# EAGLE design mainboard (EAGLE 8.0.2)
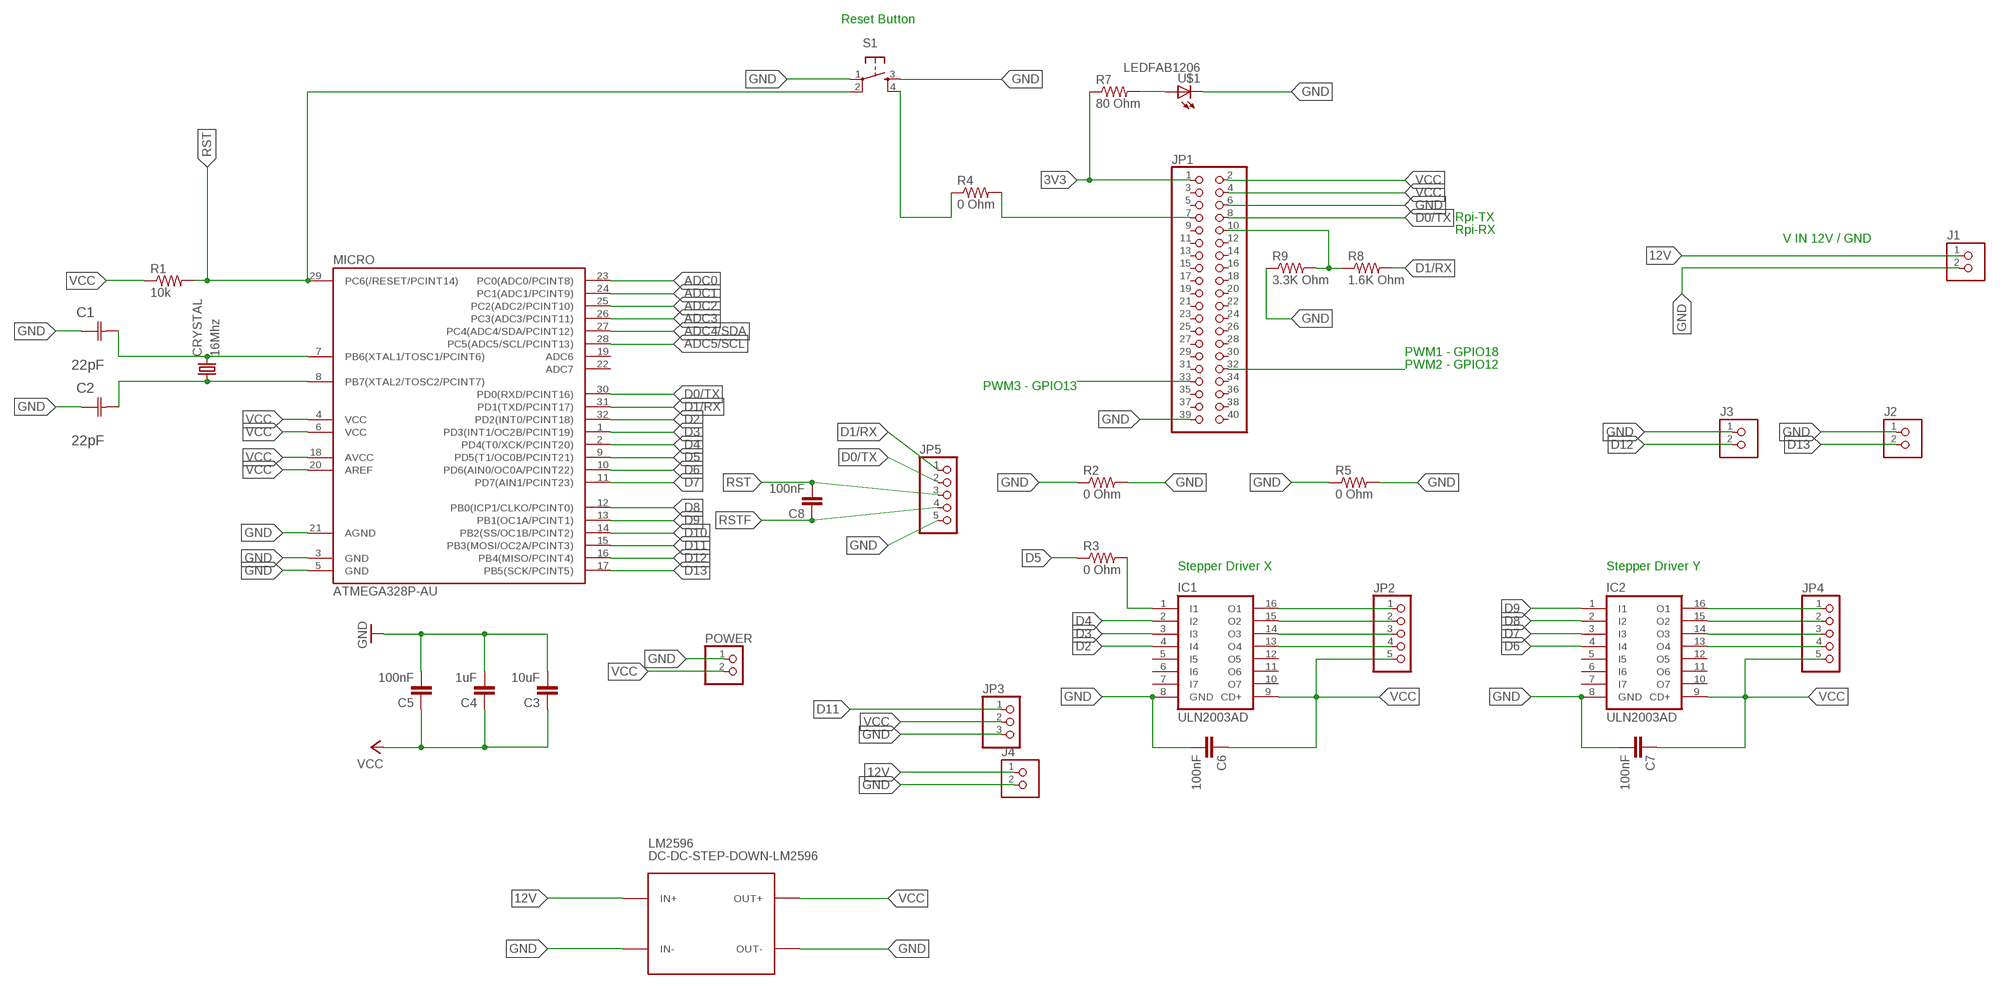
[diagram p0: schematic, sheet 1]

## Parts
C1  22pF  0612ZC225MAT2A  [CAPC3216X178N]
C2  22pF  0612ZC225MAT2A  [CAPC3216X178N]
C3  10uF  CAP1206  [1206]
C4  1uF  CAP1206  [1206]
C5  100nF  CAP1206  [1206]
C6  100nF  CAP1206  [1206]
C7  100nF  CAP1206  [1206]
C8  100nF  CAP1206  [1206]
CRYSTAL  16Mhz  CSM-7X-DU  [CSM-7X-DU]
IC1  ULN2003AD  [SO16]
IC2  ULN2003AD  [SO16]
J1  TERM-1X02-FABLAB  [ED555DS-2DS]
J2  TERM-1X02-FABLAB  [ED555DS-2DS]
J3  TERM-1X02-FABLAB  [ED555DS-2DS]
J4  TERM-1X02-FABLAB  [ED555DS-2DS]
JP1  PINHD-2X20  [2X20]
JP2  PINHD-1X5  [1X05]
JP3  PINHD-1X3  [1X03]
JP4  PINHD-1X5  [1X05]
JP5  PINHD-1X5  [1X05]
LM2596  DC-DC-STEP-DOWN-LM2596  [DC-DC-STEP-DOWN-LM2596]
MICRO  ATMEGA328P-AU  ATMEGA48/88/168-AU  [TQFP32-08]
POWER  PINHD-1X2  [1X02]
R1  10k  RESISTOR1206  [1206]
R2  0 Ohm  RES-US1206FAB  [R1206FAB]
R3  0 Ohm  RES-US1206FAB  [R1206FAB]
R4  0 Ohm  RES-US1206FAB  [R1206FAB]
R5  0 Ohm  RES-US1206FAB  [R1206FAB]
R7  80 Ohm  RES-US1206FAB  [R1206FAB]
R8  1.6K Ohm  RES-US1206FAB  [R1206FAB]
R9  3.3K Ohm  RES-US1206FAB  [R1206FAB]
S1  6MM_SWITCH6MM_SWITCH  [6MM_SWITCH]
U$1  LEDFAB1206  [LED1206FAB]

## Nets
3V3: JP1.1 R7.1
12V: J1.1 J4.1 LM2596.IN+
ADC0: MICRO.23(PC0(ADC0/PCINT8))
ADC1: MICRO.24(PC1(ADC1/PCINT9))
ADC2: MICRO.25(PC2(ADC2/PCINT10))
ADC3: MICRO.26(PC3(ADC3/PCINT11))
ADC4/SDA: MICRO.27(PC4(ADC4/SDA/PCINT12))
ADC5/SCL: MICRO.28(PC5(ADC5/SCL/PCINT13))
D0/TX: JP1.8 JP5.2 MICRO.30(PD0(RXD/PCINT16))
D1/RX: JP5.1 MICRO.31(PD1(TXD/PCINT17)) R8.2
D2: IC1.4(I4) MICRO.32(PD2(INT0/PCINT18))
D3: IC1.3(I3) MICRO.1(PD3(INT1/OC2B/PCINT19))
D4: IC1.2(I2) MICRO.2(PD4(T0/XCK/PCINT20))
D5: IC1.1(I1) MICRO.9(PD5(T1/OC0B/PCINT21)) R3.1 R3.2
D6: IC2.4(I4) MICRO.10(PD6(AIN0/OC0A/PCINT22))
D7: IC2.3(I3) MICRO.11(PD7(AIN1/PCINT23))
D8: IC2.2(I2) MICRO.12(PB0(ICP1/CLKO/PCINT0))
D9: IC2.1(I1) MICRO.13(PB1(OC1A/PCINT1))
D10: MICRO.14(PB2(SS/OC1B/PCINT2))
D11: JP3.1 MICRO.15(PB3(MOSI/OC2A/PCINT3))
D12: J3.2 MICRO.16(PB4(MISO/PCINT4))
D13: J2.2 MICRO.17(PB5(SCK/PCINT5))
GND: C1.1(C1) C2.1(C1) C3.2 C4.2 C5.2 C6.2 C7.2 IC1.8(GND) IC2.8(GND) J1.2 J2.1 J3.1 J4.2 JP1.6 JP1.39 JP3.3 JP5.5 LM2596.IN- LM2596.OUT- MICRO.3(GND) MICRO.5(GND) MICRO.21(AGND) POWER.1 R2.1 R2.2 R5.1 R5.2 R9.1 S1.1(P) U$1.2(C)
N$1: R7.2 U$1.1(A)
N$2: C1.2(C2) CRYSTAL.2 MICRO.7(PB6(XTAL1/TOSC1/PCINT6))
N$3: R4.1 S1.4(S1)
N$7: JP1.10 R8.1 R9.2
N$9: C2.2(C2) CRYSTAL.1 MICRO.8(PB7(XTAL2/TOSC2/PCINT7))
N$10: JP1.32
N$11: JP1.33
N$12: JP1.7 R4.2
N$13: IC1.16(O1) JP2.1
N$14: IC1.15(O2) JP2.2
N$15: IC1.14(O3) JP2.3
N$16: IC1.13(O4) JP2.4
N$17: S1.3(S)
N$25: IC2.16(O1) JP4.1
N$26: IC2.15(O2) JP4.2
N$27: IC2.14(O3) JP4.3
N$28: IC2.13(O4) JP4.4
RST: C8.2 JP5.3 MICRO.29(PC6(/RESET/PCINT14)) R1.2 S1.2(P1)
RSTF: C8.1 JP5.4
VCC: C3.1 C4.1 C5.1 C6.1 C7.1 IC1.9(CD+) IC2.9(CD+) JP1.2 JP1.4 JP2.5 JP3.2 JP4.5 LM2596.OUT+ MICRO.4(VCC) MICRO.6(VCC) MICRO.18(AVCC) MICRO.20(AREF) POWER.2 R1.1
Unconnected: IC1.5(I5) IC1.6(I6) IC1.7(I7) IC1.10(O7) IC1.11(O6) IC1.12(O5) IC2.5(I5) IC2.6(I6) IC2.7(I7) IC2.10(O7) IC2.11(O6) IC2.12(O5) JP1.3 JP1.5 JP1.9 JP1.11 JP1.12 JP1.13 JP1.14 JP1.15 JP1.16 JP1.17 JP1.18 JP1.19 JP1.20 JP1.21 JP1.22 JP1.23 JP1.24 JP1.25 JP1.26 JP1.27 JP1.28 JP1.29 JP1.30 JP1.31 JP1.34 JP1.35 JP1.36 JP1.37 JP1.38 JP1.40 MICRO.19(ADC6) MICRO.22(ADC7)

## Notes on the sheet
- Reset Button
- Rpi-TX
- Rpi-RX
- V IN 12V / GND
- PWM1 - GPIO18
- PWM2 - GPIO12
- PWM3 - GPIO13
- Stepper Driver X | Stepper Driver Y

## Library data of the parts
C1 C2 = AVX_By_element14_Batch_1:0612ZC225MAT2A: Capacitor 1206; MPN: 0612ZC225MAT2A; OC_FARNELL: -; OC_NEWARK: 12N3209; SUPPLIER: AVX; TOLERANCE: ±20%; VALUE: 2.2µF; VOLTAGERATING: 10V
C3-C8 = 01_SparkFun:CAP: Capacitor
CRYSTAL = 01_FAB_Hello:CSM-7X-DU: SMD CRYSTAL; OC_FARNELL: unknown; OC_NEWARK: unknown
IC1 IC2 = uln-udn:ULN2003A: DRIVER ARRAY
J1-J3 = fab:TERM-1X02: 3.5mm terminal block, 2 positions ED555-2DS as found in the fablab inventory.
J4 = fab-modd:TERM-1X02: 3.5mm terminal block, 2 positions ED555-2DS as found in the fablab inventory.
JP1 = pinhead:PINHD-2X20: PIN HEADER
JP2 JP4 JP5 = pinhead:PINHD-1X5: PIN HEADER
JP3 = pinhead:PINHD-1X3: PIN HEADER
LM2596 = diy-modules:DC-DC-STEP-DOWN-LM2596: DC/DC Step-Down Regulator based on LM2596-ADJ chip LM2596 datasheet available here: http://www.ti.com/lit/ds/symlink/lm2596.pdf Click here to find device on ebay.com
MICRO = atmega8:ATMEGA48/88/168
POWER = pinhead:PINHD-1X2: PIN HEADER
R1 = 01_SparkFun:RESISTOR: Resistor
R2-R5 R7-R9 = fab:RES-US: Resistor (US Symbol)
S1 = fab:6MM_SWITCH: OMRON SWITCH
U$1 = fab:LED: LED

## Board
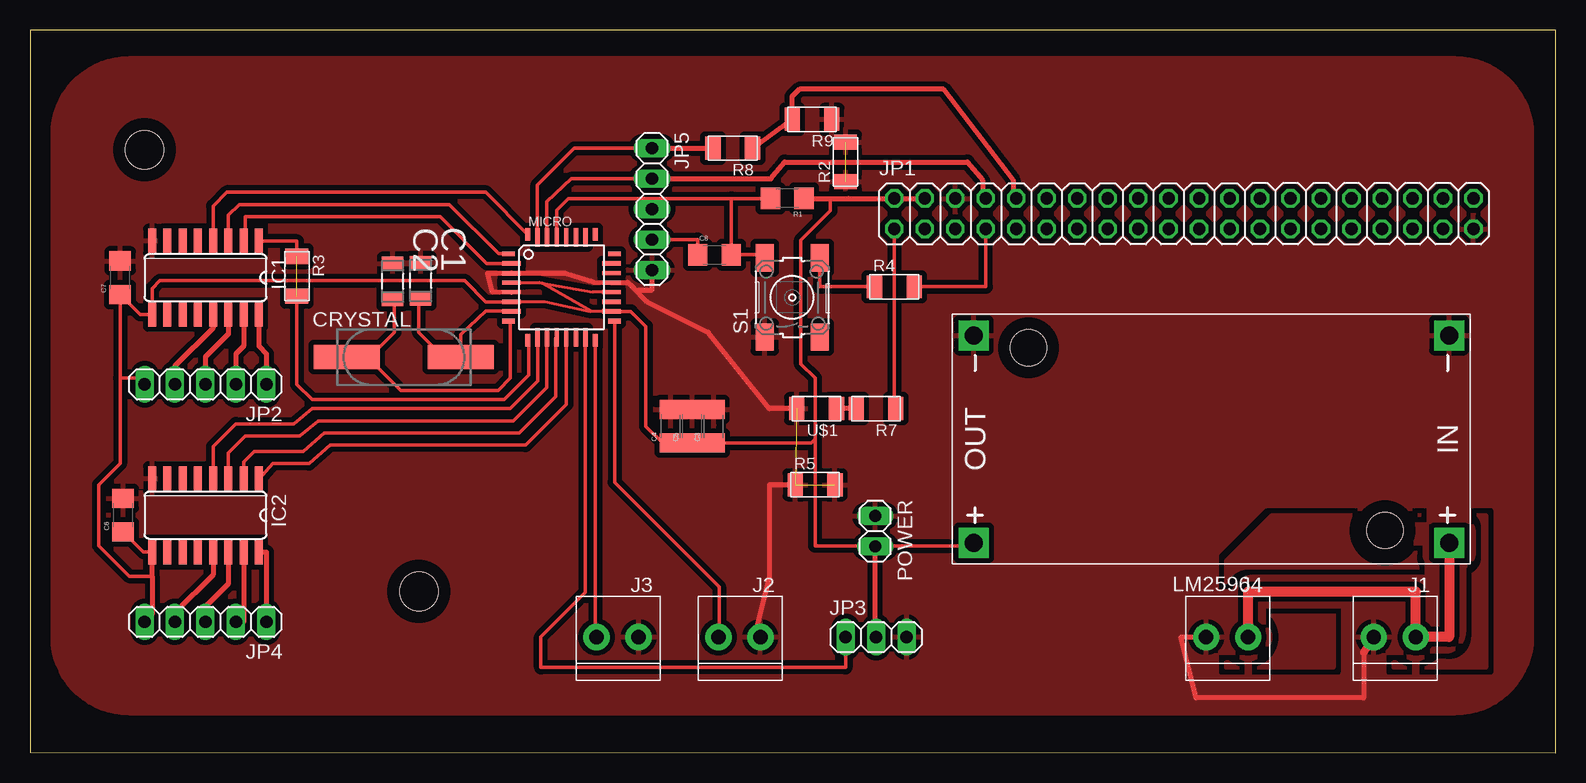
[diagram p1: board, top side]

Size 127.15 x 60.26 mm. Coordinates in mm from the lower left corner, seen from the top.
Outline: 0,0.04 127.15,0 127.15,60.26 0,60.22 0,0.04
Copper layers (1*16): Top 0.035mm / dielectric 1.5mm / Bottom 0.035mm
Design rules "default *": minimum track width 10mil, minimum drill 24mil, track to track 8mil, track to pad 8mil, pad to pad 8mil, via to via 8mil, smd to smd 8mil, copper to edge 40mil, drill to drill 8mil, minimum pad ring 10mil, minimum via ring 8mil, stop-mask expansion 4mil, vias tented up to drill 0mil, thermal gap 16mil
Holes 3.2 mm at 9.54,50.28 32.4,13.45

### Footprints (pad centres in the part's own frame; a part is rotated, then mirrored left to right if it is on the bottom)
CAPC3216X178N = smd 1.118 x 1.803: 1 -1.499,0; 2 1.499,0
1206 = smd 1.6 x 1.8: 1 -1.4,0; 2 1.4,0
CSM-7X-DU = smd 5.5 x 2: 1 -4.75,0; 2 4.75,0
SO16 = smd 0.66 x 2.032: 1 -4.445,-3.073; 2 -3.175,-3.073; 3 -1.905,-3.073; 4 -0.635,-3.073; 5 0.635,-3.073; 6 1.905,-3.073; 7 3.175,-3.073; 8 4.445,-3.073; 9 4.445,3.073; 10 3.175,3.073; 11 1.905,3.073; 12 0.635,3.073; 13 -0.635,3.073; 14 -1.905,3.073; 15 -3.175,3.073; 16 -4.445,3.073
ED555DS-2DS = drill 1.2 pad 2.184: 1 1.8,0; 2 -1.7,0
2X20 = drill 1.016 octagon: 1 -24.13,-1.27; 2 -24.13,1.27; 3 -21.59,-1.27; 4 -21.59,1.27; 5 -19.05,-1.27; 6 -19.05,1.27; 7 -16.51,-1.27; 8 -16.51,1.27; 9 -13.97,-1.27; 10 -13.97,1.27; 11 -11.43,-1.27; 12 -11.43,1.27; 13 -8.89,-1.27; 14 -8.89,1.27; 15 -6.35,-1.27; 16 -6.35,1.27; 17 -3.81,-1.27; 18 -3.81,1.27; 19 -1.27,-1.27; 20 -1.27,1.27; 21 1.27,-1.27; 22 1.27,1.27; 23 3.81,-1.27; 24 3.81,1.27; 25 6.35,-1.27; 26 6.35,1.27; 27 8.89,-1.27; 28 8.89,1.27; 29 11.43,-1.27; 30 11.43,1.27; 31 13.97,-1.27; 32 13.97,1.27; 33 16.51,-1.27; 34 16.51,1.27; 35 19.05,-1.27; 36 19.05,1.27; 37 21.59,-1.27; 38 21.59,1.27; 39 24.13,-1.27; 40 24.13,1.27
1X05 = drill 1.016 long: 1 -5.08,0; 2 -2.54,0; 3 0,0; 4 2.54,0; 5 5.08,0
1X03 = drill 1.016 long: 1 -2.54,0; 2 0,0; 3 2.54,0
DC-DC-STEP-DOWN-LM2596 = drill 1.5 pad 2.5 square: IN+ -19.812,8.636; IN- -19.812,-8.636; OUT+ 19.812,8.636; OUT- 19.812,-8.636 | hole 3: -14.478,7.62; 15.24,-7.62
TQFP32-08 = smd 1.016 x 0.406: 1 -4.42,2.8; 8 -4.42,-2.8; 17 4.42,-2.8; 24 4.42,2.8 | smd 1.524 x 0.356: 2 -4.166,2; 3 -4.166,1.2; 4 -4.166,0.4; 5 -4.166,-0.4; 6 -4.166,-1.2; 7 -4.166,-2; 18 4.166,-2; 19 4.166,-1.2; 20 4.166,-0.4; 21 4.166,0.4; 22 4.166,1.2; 23 4.166,2 | smd 0.406 x 1.016: 9 -2.8,-4.42; 16 2.8,-4.42; 25 2.8,4.42; 32 -2.8,4.42 | smd 0.356 x 1.524: 10 -2,-4.166; 11 -1.2,-4.166; 12 -0.4,-4.166; 13 0.4,-4.166; 14 1.2,-4.166; 15 2,-4.166; 26 2,4.166; 27 1.2,4.166; 28 0.4,4.166; 29 -0.4,4.166; 30 -1.2,4.166; 31 -2,4.166
1X02 = drill 1.016 long: 1 -1.27,0; 2 1.27,0
R1206FAB = smd 1.27 x 1.905: 1 -1.651,0; 2 1.651,0
6MM_SWITCH = smd 2.286 x 1.524: 1 -3.302,2.286; 2 3.302,2.286; 3 -3.302,-2.286; 4 3.302,-2.286
LED1206FAB = smd 1.27 x 1.905: 1 -1.651,0; 2 1.651,0

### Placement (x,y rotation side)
C1  32.55,39.36 270 top
C2  30.22,39.31 270 top
C3  56.99,27.22 90 top
C4  53.38,27.22 90 top
C5  55.19,27.22 90 top
C6  7.76,19.8 90 top
C7  7.51,39.61 90 top
C8  57.04,41.52 0 top
CRYSTAL  31.16,32.98 0 top
IC1  14.62,39.61 180 top
IC2  14.62,19.8 180 top
J1  113.68,9.64 0 top
J2  59.07,9.64 0 top
J3  48.91,9.64 0 top
J4  99.71,9.64 0 top
JP1  96.16,44.95 0 top
JP2  14.62,30.72 180 top
JP3  70.5,9.64 0 top
JP4  14.62,10.91 180 top
JP5  51.83,45.33 270 top
LM2596  98.44,26.15 180 top
MICRO  44.29,38.8 0 top
POWER  70.43,18.47 270 top
R1  63.1,46.22 180 top
R2  67.96,49.26 90 top
R3  22.24,39.74 270 top
R4  72.03,38.85 0 top
R5  65.42,22.34 0 top
R7  70.5,28.69 180 top
R8  58.56,50.41 180 top
R9  65.17,52.82 180 top
S1  63.52,37.96 90 top
U$1  65.55,28.69 180 top

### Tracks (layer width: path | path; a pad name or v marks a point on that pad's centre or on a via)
3V3
  Top 0.305: JP1.1 72.03,28.82 R7.1
12V
  Top 0.813: LM2596.IN+ 118.25,9.64 J1.1 115.48,13.45 101.51,13.45 J4.1
D0/TX
  Top 0.305: JP5.2 45.1,47.87 43.07,45.96 43.07,42.99 MICRO.30 | 51.96,47.87 52.72,48.37 52.21,47.87 51.96,47.87
  Top 0.406: JP5.2 51.96,47.87 61.74,47.87 62.88,49.26 78.12,49.26 79.39,47.74 79.39,46.47 JP1.8
D1/RX
  Top 0.305: MICRO.31 42.29,47.34 45.36,50.41 51.45,50.41 | 51.45,50.41 52.72,50.03 52.34,50.41 JP5.1 51.45,50.41
  Top 0.406: JP5.1 R8.2
D2
  Top 0.305: MICRO.32 37.99,46.72 16.4,46.72 15.26,45.58 IC1.4
D3
  Top 0.305: IC1.3 16.53,44.82 17.42,45.71 34.94,45.71 39.05,41.6 MICRO.1
D4
  Top 0.305: MICRO.2 38.07,40.8 34.18,44.69 17.92,44.69 17.92,42.81 IC1.2
D5  (1 unrouted)
  Top 0.305: R3.1 22.24,42.66 19.09,42.66 IC1.1 | R3.2 22.24,30.72 23.51,29.45 39.51,29.45 41.55,31.48 41.55,34.32 MICRO.9
D6
  Top 0.305: IC2.4 15.26,25.51 17.16,27.42 21.99,27.42 23.51,28.69 40.02,28.69 42.31,30.98 42.31,34.62 MICRO.10
D7
  Top 0.305: IC2.3 16.53,25.01 17.92,26.4 22.5,26.4 24.02,27.67 40.28,27.67 43.07,30.47 43.07,34.62 MICRO.11
D8
  Top 0.305: IC2.2 17.8,24.24 18.69,25.13 22.75,25.13 24.53,26.66 40.78,26.66 43.83,29.71 43.83,34.58 MICRO.12
D9
  Top 0.305: IC2.1 19.09,22.85 20.21,24.12 23.26,24.12 25.04,25.64 41.29,25.64 44.69,29.04 MICRO.13
D11
  Top 0.305: MICRO.15 46.29,13.37 42.56,9.64 42.56,7.1 67.96,7.1 JP3.1
D12
  Top 0.305: MICRO.16 47.09,9.76 J3.2
D13
  Top 0.305: MICRO.17 48.71,22.54 57.42,13.83 57.42,9.69 J2.2
GND  (3 unrouted)
  Top 0.305: MICRO.21 | C4.2 C5.2 C3.2
  Top 0.406: MICRO.5 38.5,38.47 38.12,39.99 MICRO.3 44.59,39.99 47.01,39.23 MICRO.21 | MICRO.21 49.8,39.23 49.87,39.17 | 50.18,38.85 49.87,39.17 | 50.18,38.85 50.44,38.6 51.83,38.6 JP5.5 | 111.14,8.37 111.14,4.56 97.17,4.56 95.9,9.64 J4.2 | MICRO.21 49.87,39.17 | U$1.2 61.61,28.69 56.53,35.04 51.45,37.58 50.18,38.85 | R5.1 61.61,22.34 61.61,14.72 60.34,9.64 61.61,9.64
  Top 0.61: J1.2 111.14,8.37
  pour Top (isolate 0.432, rank 3): 118.76,3.29 8.27,3.29 arc-90 1.92,9.64 1.92,51.55 arc-90 8.27,57.9 118.76,57.9 arc-90 125.11,51.55 125.11,9.64 arc-90
N$1
  Top 0.406: R7.2 U$1.1
N$2
  Top 0.305: C1.2 32.4,37.58 32.4,35.04 34.59,32.85 CRYSTAL.2 35.91,34.87 37.99,36.82 40.11,36.82 MICRO.7
N$3
  Top 0.305: S1.4 65.8,38.85 R4.1
N$7
  Top 0.406: R8.1 R9.2 63.52,54.72 64.15,55.36 76.09,55.36 81.93,47.74 81.93,46.47 JP1.10
N$9
  Top 0.305: C2.2 30.37,37.53 30.37,35.04 28.18,32.85 CRYSTAL.1 28.24,32.85 30.88,30.21 39.01,30.21 40.02,31.23 40.02,35.85 MICRO.8
N$12
  Top 0.305: JP1.7 79.65,38.85 R4.2
N$13
  Top 0.406: IC1.16 19.07,33.9 19.7,33.26 JP2.1
N$14
  Top 0.406: IC1.15 17.8,33.9 17.16,33.26 JP2.2
N$15
  Top 0.406: IC1.14 16.53,34.91 14.62,33.01 JP2.3
N$16
  Top 0.406: IC1.13 15.26,35.42 12.08,32.25 JP2.4
N$18
  pour Top (isolate 1.422, rank 2, no thermals): 99.71,7.1 99.71,15.99 103.52,19.8 121.3,19.8 121.3,7.1 113.68,7.1 113.68,12.18 108.6,12.18 108.6,7.1
N$25
  Top 0.406: IC2.16 19.7,16.73 JP4.1
N$26
  Top 0.406: IC2.15 17.8,10.91 JP4.2
N$27
  Top 0.406: IC2.14 16.53,14.08 14.62,12.18 JP4.3
N$28
  Top 0.406: IC2.13 15.26,14.85 12.08,11.67 JP4.4
RST
  Top 0.305: MICRO.29 43.89,45.26 44.85,46.22 50.94,46.22 | 52.72,46.22 50.94,46.22 | 50.94,46.22 JP5.3 52.72,46.22 | S1.2 60.98,41.52 C8.2 58.44,46.22 | 52.72,46.22 58.44,46.22 | 58.44,46.22 62.2,46.22 R1.2
RSTF
  Top 0.305: JP5.4 55.64,42.79 C8.1
VCC
  Top 0.254: MICRO.20 47.85,38.4 47.85,38.42 46.88,38.42 42.65,39.17 | MICRO.4 42.47,39.21 42.65,39.17 | 40.81,37.61 42.89,37.61 46.71,36.8 MICRO.18 | 48.46,36.81 MICRO.18 46.83,36.8 42.65,39.17
  Top 0.305: MICRO.18 | MICRO.20 47.85,38.42 | 48.46,36.77 MICRO.18 | 40.81,37.61 MICRO.6 40.12,37.58 37.99,37.58 36.21,39.36 10.81,39.36 10.18,38.72 IC1.9 9.18,36.54 C7.1 7.51,31.23 | 48.46,36.81 MICRO.18 | IC2.9 9.44,16.73 C6.1 | 7.51,31.23 7.51,24.12 5.73,22.34 5.73,17.26 8.27,14.72 10.18,14.72 | 7.51,31.23 9.03,31.23 JP2.5 | MICRO.18 50.07,36.8 51.33,35.55 51.33,27.2 52.72,25.81 53.97,25.81 54,25.78 53.42,25.78 C4.1 C5.1 C3.1 65.09,25.82 65.42,26.15 | 65.42,26.15 65.42,31.23 64.25,32.41 64.25,42.75 66.69,45.2 66.69,46.13 R1.1 | 65.42,17.26 65.42,26.15 | LM2596.OUT+ 78.38,17.26 70.43,17.26 | 70.43,17.26 65.42,17.26 | 65.42,17.25 65.42,17.26 | 70.43,17.26 POWER.2 70.43,9.64
  Top 0.406: IC2.9 10.18,14.72 10.18,11.54 JP4.5 | JP1.4 JP1.2 68.21,46.22 R1.1 | JP3.2 70.43,9.64 POWER.2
